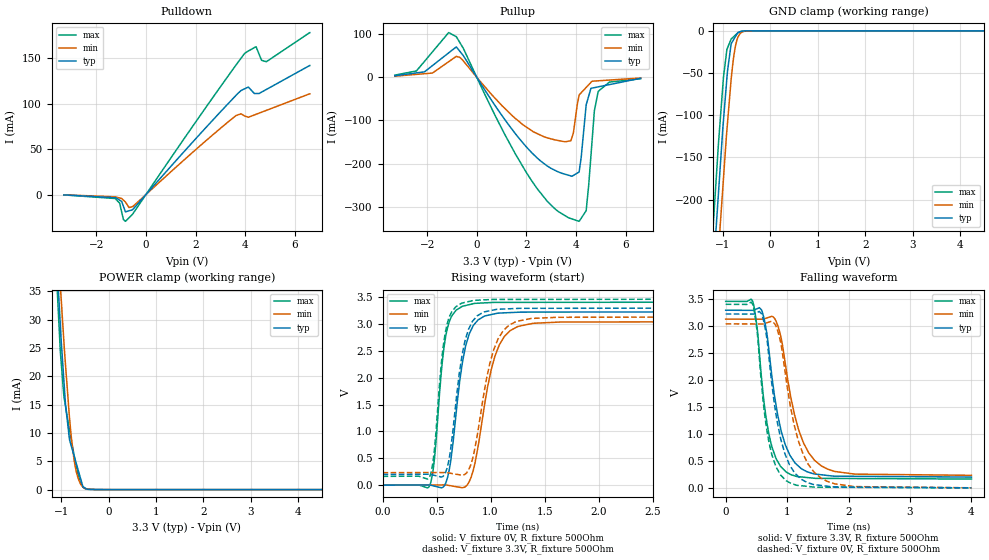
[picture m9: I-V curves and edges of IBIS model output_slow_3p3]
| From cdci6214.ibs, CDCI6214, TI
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|   output_slow_3p3 Model
[Model]   output_slow_3p3
Model_type   3-state
Polarity   Non-Inverting
Vmeas = 1.65
Vref = 0
Cref = 1pF
Rref = 100000
|   typ   min   max
C_comp   5.349E-12   5.278E-12   5.416E-12
|  Where Nom  PVT is Nominal Process, 3.3V,   32C
|   Fast PVT is Strong Process,  3.465V, -35C
|   Slow PVT is Weak Process,   3.135V,  110C
[Voltage Range]   3.3   3.135   3.465
|Junction Temperature
[Temperature Range]   32   110   -35
[Pullup Reference]   3.3   3.135   3.465
[Pulldown Reference]   0   0   0
[Power Clamp Reference]   3.3   3.135   3.465
[GND Clamp Reference]   0   0   0
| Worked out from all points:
|   slope of the pulldown table from 0 to 0.495 V, typ, clamps not added: 32.3 ohm
|   slope of the pullup table from 0 to 0.495 V, typ, clamps not added: 11.1 ohm
|   GND clamp passes 1 mA (typ) near -0.64 V on its own axis
|   POWER clamp passes 1 mA (typ) near -0.56 V on its own axis
|   falling waveform, V_fixture 3.3V, R_fixture 500Ohm: 20-80 % time 273ps typ, 339ps min, 212ps max; typ from 3.3 V to 0.2 V
|   rising waveform, V_fixture 0V, R_fixture 500Ohm: 20-80 % time 125ps typ, 173ps min, 92.1ps max; typ from 0 V to 3.23 V
|   rising waveform, V_fixture 3.3V, R_fixture 500Ohm: 20-80 % time 123ps typ, 169ps min, 90.8ps max; typ from 0.2 V to 3.3 V
|   falling waveform, V_fixture 0V, R_fixture 500Ohm: 20-80 % time 271ps typ, 336ps min, 211ps max; typ from 3.23 V to 0 V
[Pulldown]
|   Voltage   I(typ)   I(min)   I(max)
-3.3V     -335.9uA   -281.5uA   -389.7uA
-1.243V   -3.448mA   -2.514mA   -4.326mA
-1.06V    -6.073mA   -3.74mA    -9.302mA
-906mV    -12.91mA   -6.122mA   -27.55mA
-824.9mV  -19mA      -8.207mA   -29.41mA
-531.3mV  -16.44mA   -13.18mA   -21.35mA
3.553V    106.9mA    85.33mA    139.6mA
3.971V    116.3mA    86.5mA     155.2mA
4.433V    111.1mA    88.25mA    162.7mA
4.659V    112.7mA    90.61mA    147.7mA
4.85V     115.6mA    92.61mA    146.1mA
6.6V      142mA      110.9mA    178.2mA
[GND Clamp]
|   Voltage   I(typ)   I(min)   I(max)
-3.3V     -2.319A    -2.383A    -2.268A
-1.251V   -332.1mA   -407.3mA   -272.1mA
-1.148V   -238.6mA   -314mA     -181.9mA
-1.055V   -160.9mA   -229.9mA   -105.5mA
-986.2mV  -105.4mA   -174.3mA   -54.58mA
-903.2mV  -48.1mA    -109.9mA   -20.47mA
-825mV    -15.26mA   -57.33mA   -9.728mA
-793.7mV  -12.32mA   -40.72mA   -8.068mA
-738.3mV  -7.106mA   -19.15mA   -5.15mA
-682.4mV  -1.92mA    -7.571mA   -2.61mA
-336.3mV  -2.307uA   -4.808uA   -31.76uA
6.6V      0A         0A         0A
[Pullup]
|   Voltage   I(typ)   I(min)   I(max)
-3.3V     3.521mA    2.458mA    4.852mA
-2.106V   12.54mA    8.23mA     36.78mA
-1.131V   56.56mA    36.03mA    103.6mA
-824.9mV  70.35mA    48.34mA    94.15mA
1.576V    -132.3mA   -96.37mA   -179.8mA
2.823V    -204.9mA   -140.1mA   -286.1mA
3.792V    -228.7mA   -147.1mA   -327.5mA
4.118V    -219.7mA   -43.07mA   -333.8mA
4.406V    -64.22mA   -23.64mA   -309.2mA
4.737V    -24.06mA   -8.797mA   -77.97mA
4.889V    -22.28mA   -8.22mA    -32.92mA
6.6V      -2.365mA   -1.748mA   -3.522mA
[POWER Clamp]
|   Voltage   I(typ)   I(min)   I(max)
-3.3V     442.7mA    387.3mA    532.5mA
-1.124V   45.42mA    50.88mA    42.06mA
-1.059V   35.33mA    41.4mA     31.21mA
-1.006V   27.13mA    34.45mA    23.12mA
-942.7mV  19.22mA    26.11mA    16.43mA
-909.1mV  15.04mA    22.05mA    14.73mA
-825mV    8.811mA    12.69mA    10.47mA
-751.1mV  6.646mA    6.651mA    7.139mA
-638.3mV  3.338mA    1.869mA    2.592mA
-541.8mV  512.2uA    442.3uA    471.7uA
-471.4mV  154.4uA    118.1uA    66.78uA
6.6V      0A         0A         0A
[Ramp]
R_load = 500
|   typ   min   max
dV/dt_r   1.93765/1.24072e-10   1.82706/1.71061e-10   2.04591/9.14201e-11
dV/dt_f   1.8599/2.72171e-10   1.74107/3.37211e-10   1.98068/2.11191e-10
[Falling Waveform]
V_fixture = 3.3V
V_fixture_min = 3.135V
V_fixture_max = 3.465V
R_fixture = 500Ohm
C_fixture = 0F
|   Time   V(typ)   V(min)   V(max)
0s        3.3V       3.134V     3.465V
439.4ps   3.298V     3.133V     3.467V
515.8ps   3.331V     3.133V     2.938V
581.5ps   3.309V     3.133V     2.068V
727.8ps   2.316V     3.178V     874.5mV
849.2ps   1.34V      3.012V     486.3mV
982.8ps   768.7mV    2.214V     295.5mV
1.191ns   397.7mV    1.066V     206.9mV
1.561ns   242.8mV    405mV      176mV
4ns       200mV      232.6mV    163.8mV
[Rising Waveform]
V_fixture = 0V
V_fixture_min = 0V
V_fixture_max = 0V
R_fixture = 500Ohm
C_fixture = 0F
|   Time   V(typ)   V(min)   V(max)
0s        316.6uV    1.239mV    45.45uV
436.4ps   4.217mV    3.543mV    -8.488mV
479.8ps   -17.01mV   3.772mV    476.9mV
584.8ps   39.39mV    4.326mV    2.773V
631.3ps   452.8mV    -10.76mV   3.111V
736.8ps   2.249V     -48.11mV   3.33V
838.2ps   2.969V     265.5mV    3.379V
1.041ns   3.193V     2.408V     3.404V
1.251ns   3.221V     2.955V     3.405V
4ns       3.23V      3.046V     3.41V
[Rising Waveform]
V_fixture = 3.3V
V_fixture_min = 3.135V
V_fixture_max = 3.465V
R_fixture = 500Ohm
C_fixture = 0F
|   Time   V(typ)   V(min)   V(max)
0s        200mV      232.6mV    163.8mV
436.4ps   203.9mV    234.8mV    156.3mV
476.8ps   184.3mV    235.1mV    595.4mV
581.8ps   228.9mV    235.6mV    2.85V
626.3ps   609.5mV    222.4mV    3.171V
732.8ps   2.38V      185.9mV    3.389V
829.2ps   3.039V     460mV      3.435V
1.028ns   3.264V     2.518V     3.459V
1.237ns   3.291V     3.049V     3.46V
4ns       3.3V       3.134V     3.465V
[Falling Waveform]
|Gnd
V_fixture = 0V
V_fixture_min = 0V
V_fixture_max = 0V
R_fixture = 500Ohm
C_fixture = 0F
|   Time   V(typ)   V(min)   V(max)
0s        3.23V      3.046V     3.41V
439.4ps   3.228V     3.045V     3.411V
513.8ps   3.259V     3.045V     2.885V
581.5ps   3.236V     3.045V     1.953V
726.8ps   2.187V     3.089V     730.9mV
872.2ps   1.043V     2.816V     281.9mV
981.8ps   584.8mV    2.034V     135.2mV
1.182ns   211.4mV    877.4mV    44.92mV
1.553ns   44.69mV    181mV      12.05mV
4ns       316.4uV    1.24mV     46.88uV
